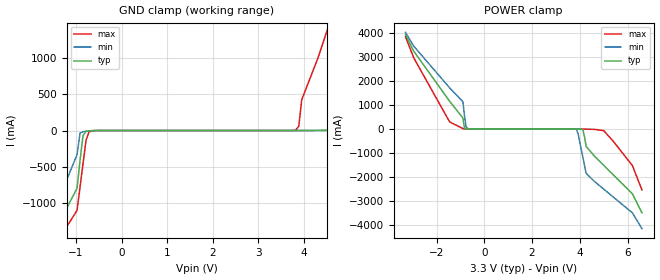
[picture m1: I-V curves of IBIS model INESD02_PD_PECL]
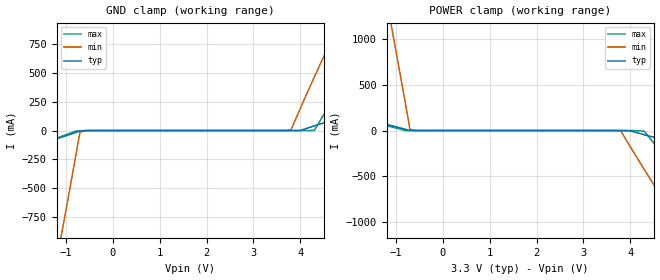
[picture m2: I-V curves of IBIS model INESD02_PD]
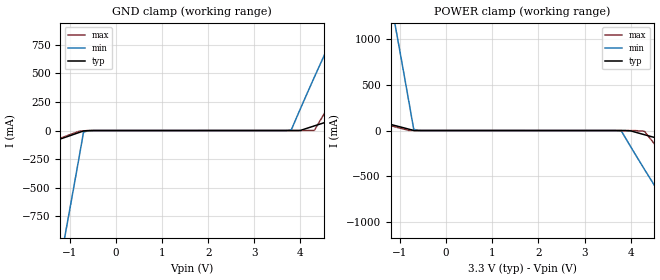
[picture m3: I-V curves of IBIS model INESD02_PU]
|   This file is an IBIS representation of the   |
|   Integrated Device Technology, Inc.   |
|   ICS874001I-02   |
|   PCI EXPRESS JITTER ATTENUATOR   |
[IBIS Ver]   4.1
[File name]   874001i_02.ibs
[File Rev]   1.0
[Date]   14 Sep 2011
[Source]   Originated at Integrated Device Technology, Inc.
[Disclaimer]
IDT hereby grants the user of this IBIS model a non-exclusive,
nontransferable license to use this IBIS model under the following terms.
Before using this IBIS model, the user should read this license.
If the user does not accept these terms,  the IBIS model should be
returned to IDT within 30 days.
   The user is granted this license only to use the IBIS model and
is not granted rights to sell, load, rent, lease or license the IBIS
model in whole or in part, or in modified form to anyone other than
user. User may modify the IBIS model to suit its specific
applications but rights to derivative works and such modifications
shall belong to IDT.
   This IBIS model is provided on an "AS IS" basis and IDT makes
absolutely no warranty with respect to the information contained
herein. IDT DISCLAIMS AND CUSTOMER WAIVES ALL WARRANTIES, EXPRESS
OR IMPLIED, INCLUDING WARRANTIES OF MERCHANTABILITY OR FITNESS FOR
A PARTICULAR PURPOSE. The entire risk as to quality and performance
is with the Customer. ACCORDINGLY, IN NO EVENT SHALL THE COMPANY BE
LIABLE FOR ANY DAMAGES, WHETHER IN CONTRACT OR TORT,INCLUDING ANY
LOST PROFITS OR OTHER INCIDENTAL, CONSEQUENTIAL, EXEMPLARY, OR
PUNITIVE DAMAGES ARISING OUT OF THE USE OR APPLICATION OF THE IBIS
model provided in this package. Further, IDT reserves the right to
make changes without notice to any product herein to improve
reliability, function, or design. IDT does not convey any license
under patent rights or any other intellectual property rights,
including those of third parties.
   IDT is not obligated to provide maintenance or support
for the licensed IBIS model.
[Copyright]   Copyright 2011 by Integrated Device Technology, Inc.
[Component]   ICS874001GI-02
[Manufacturer] Integrated Device Technology, Inc.
[Package]
|TSSOP 20 Lead
|   typ   min   max
R_pkg   51.85m   41.1m   62.6m
L_pkg   1.568nH   0.734nH   2.401nH
C_pkg   0.221pF   0.068pF   0.373pF
[Pin] signal_name   model_name   R_pin   L_pin   C_pin
1  PLL_SEL   INESD02_PD_PECL   62.6m   2.401n   0.373p
2  nc   nc   57.23m   1.985n   0.297p
3  nc   nc   51.85m   1.568n   0.221p
4  nc   nc   46.78m   1.151n   0.145p
5  MR   INESD02_PD_PECL   41.1m   0.734n   0.068p
6  BW_SEL   INESD02_PD   41.1m   0.734n   0.068p
7  F_SEL1   INESD02_PU   46.78m   1.151n   0.145p
8  VDDA   POWER   51.85m   1.568n   0.221p
9  F_SEL0   INESD02_PD   57.23m   1.985n   0.297p
10 VDD   POWER   62.6m   2.401n   0.373p
11 OE   INESD02_PU   62.6m   2.401n   0.373p
12 CLK   INESD02_PD_PECL   57.23m   1.985n   0.297p
13 nCLK   INESD02_PU_PECL   51.85m   1.568n   0.221p
14 GND   GND   46.78m   1.151n   0.145p
15 nc   nc   41.1m   0.734n   0.068p
16 nc   nc   41.1m   0.734n   0.068p
17 nQ   ONLVDS03_LVDS01_   46.78m   1.151n   0.145p
18 Q   ONLVDS03_LVDS01_   51.85m   1.568n   0.221p
19 VDDO   POWER   57.23m   1.985n   0.297p
20 nc   nc   62.6m   2.401n   0.373p
[Diff Pin]  inv_pin  vdiff tdelay_typ tdelay_min  tdelay_max
12   13   0.15   0   0   0
18   17   NA   0   0   0
| Models and submodels in the file (5): INESD02_PD_PECL (Input), INESD02_PD (Input), INESD02_PU (Input), INESD02_PU_PECL (Input), ONLVDS03_LVDS01_ (Output)
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[Model]   INESD02_PD_PECL
Model_type  Input
Polarity   Non-Inverting
Vinl = 0.8V
Vinh = 2.0V
|   typ   min   max
C_comp   2pF   1.5pF   2.5pF
|   typ   min   max
[Voltage range]  3.3V   3.135V   3.465V
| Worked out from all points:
|   GND clamp passes 1 mA (typ) near -0.59 V on its own axis
|   POWER clamp passes 1 mA (typ) near -0.70 V on its own axis
[GND_clamp]
-3.3V     -3.894A    -4.294A    -3.674A
-1.6V     -1.569A    -1.322A    -1.74A
-974.8mV  -794.1mA   -331.5mA   -1.096A
-843.4mV  -68.33mA   -15.34mA   -452.9mA
-646.5mV  -1.912mA   -4.151mA   -2.665mA
3.818V    89.38uA    70.49uA    7.198mA
3.95V     342.2uA    75.94uA    423.8mA
4.6V      7.437mA    165.5uA    1.553A
4.9V      78.32mA    440.9uA    2.118A
5.5V      1.293A     2.769mA    3.249A
6.25V     2.651A     112.4mA    4.38A
6.6V      3.331A     896.1mA    4.946A
[POWER_clamp]
-3.3V     3.923A     4.017A     3.838A
-2.95V    3.23A      3.44A      2.951A
-1.45V    1.149A     1.709A     289.6mA
-896.9mV  456.5mA    1.133A     15.4mA
-762.9mV  4.223mA    91.07mA    1.486mA
-695.9mV  792.2uA    10.73mA    555.6uA
3.861V    -556.7uA   -26.14mA   -39.45uA
4.129V    -41.85mA   -1.19A     -4.904mA
4.263V    -724.2mA   -1.847A    -12.04mA
5V        -1.514A    -2.505A    -71.38mA
6.2V      -2.701A    -3.492A    -1.525A
6.6V      -3.492A    -4.151A    -2.536A
[Model]   INESD02_PD
Model_type   Input
Polarity   Non-Inverting
Vinl = 0.8V
Vinh = 2.0V
|   typ   min   max
C_comp   2pF   1.5pF   2.5pF
|   typ   min   max
[Voltage range]   3.3V   3.135V   3.465V
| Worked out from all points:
|   GND clamp passes 1 mA (typ) near -0.60 V on its own axis
|   POWER clamp passes 1 mA (typ) near -0.70 V on its own axis
[GND_clamp]
|Voltage   I (typ)   I (min)   I (max)
-3.3V     -332.3mA   -5.292A    -346.3mA
-2.2V     -203.6mA   -3.226A    -207.3mA
-1.1V     -59.83mA   -918.6mA   -51.9mA
-1V       -45.96mA   -695.9mA   -36.91mA
-700mV    -3.491mA   -14.25mA   -2.553mA
-500mV    -180.1uA   -382.8uA   -57.92uA
3.8V      83.75uA    4.893mA    57.37uA
4V        862uA      192.6mA    61.17uA
4.3V      40.69mA    467.1mA    1.452mA
4.8V      104.5mA    906.7mA    336.6mA
5.7V      211.5mA    1.644A     899.1mA
6.6V      309.2mA    2.318A     1.413A
[Power_clamp]
|Voltage   I (typ)   I (min)   I (max)
-3.3V     309.2mA    6.635A     293.4mA
-1.1V     53.7mA     1.148A     39.81mA
-1V       40.69mA    868.5mA    26.9mA
-800mV    14.27mA    301.3mA    677.5uA
-700mV    862uA      13.32mA    132.7uA
-500mV    83.75uA    187.9uA    60.1uA
3.8V      -180.1uA   -6.224mA   -5.27uA
4V        -3.491mA   -176.5mA   -129.9uA
4.3V      -45.96mA   -425.6mA   -8.439mA
5.2V      -165.9mA   -1.129A    -564.9mA
6.2V      -287.1mA   -1.84A     -1.127A
6.6V      -332.3mA   -2.105A    -1.336A
[Model]   INESD02_PU
Model_type   Input
Polarity   Non-Inverting
Vinl = 0.8V
Vinh = 2.0V
|   typ   min   max
C_comp   2pF   1.5pF   2.5pF
|   typ   min   max
[Voltage range]   3.3V   3.135V   3.465V
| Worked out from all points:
|   GND clamp passes 1 mA (typ) near -0.59 V on its own axis
|   POWER clamp passes 1 mA (typ) near -0.70 V on its own axis
[GND_clamp]
|Voltage   I (typ)   I (min)   I (max)
-3.3V     -332.3mA   -5.292A    -346.4mA
-2.2V     -203.6mA   -3.226A    -207.3mA
-1.1V     -59.89mA   -918.7mA   -51.95mA
-1V       -46.02mA   -696mA     -36.96mA
-700mV    -3.555mA   -14.33mA   -2.605mA
-500mV    -244.4uA   -459.2uA   -110.2uA
3.8V      19.46uA    4.817mA    5.058uA
4V        797.8uA    192.5mA    8.864uA
4.3V      40.63mA    467mA      1.399mA
4.8V      104.4mA    906.6mA    336.6mA
5.7V      211.4mA    1.644A     899.1mA
6.6V      309.2mA    2.318A     1.413A
[Power_clamp]
|Voltage   I (typ)   I (min)   I (max)
-3.3V     309.2mA    6.635A     293.4mA
-1.1V     53.64mA    1.148A     39.76mA
-1V       40.63mA    868.5mA    26.85mA
-800mV    14.21mA    301.2mA    625.1uA
-700mV    797.8uA    13.24mA    80.41uA
-500mV    19.46uA    111.5uA    7.794uA
3.8V      -244.4uA   -6.3mA     -57.58uA
4V        -3.555mA   -176.6mA   -182.3uA
4.3V      -46.02mA   -425.6mA   -8.491mA
5.2V      -166mA     -1.129A    -565mA
6.2V      -287.2mA   -1.84A     -1.127A
6.6V      -332.3mA   -2.105A    -1.336A
